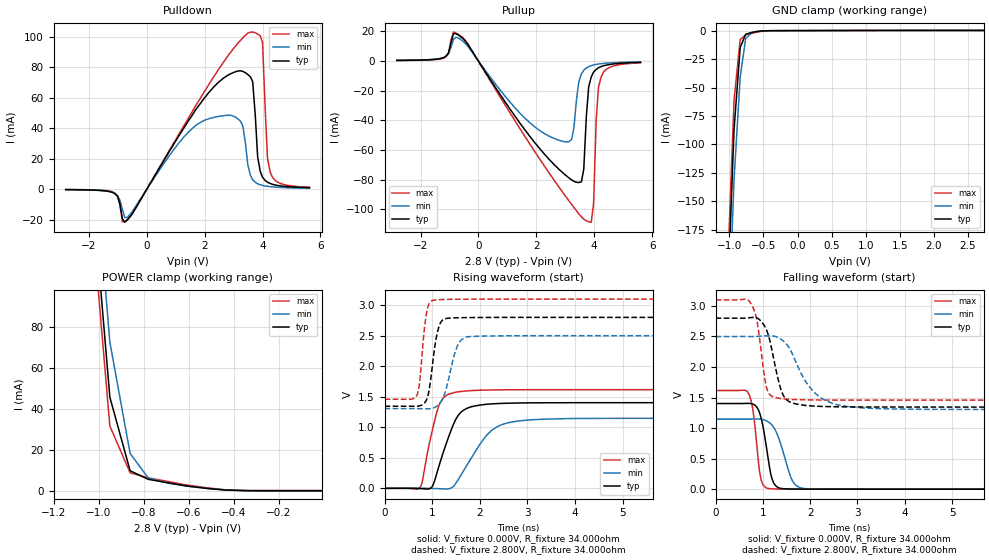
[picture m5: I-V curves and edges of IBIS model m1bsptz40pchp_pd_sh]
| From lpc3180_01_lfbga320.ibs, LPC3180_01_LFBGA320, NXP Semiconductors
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| |   Rev 0.20 IBIS Model Design Automation Generation   |
| |   N O N - S I L I C O N   C O R R E L A T E D   |
| |   This IBIS [Model] is pre-Beta tactical support   |
| |  Note: this IBIS [Model] contains clamp curves generated   |
| |   through simulation which should not be relied upon   |
| mem1bsptz40pchp
|   Bidirectional Pad 2.8
|   3state Output
|   Plain Input
|   1ns Slew Rate control
|   CMOS
| Pull Down Mode (p1=1, p2=1)
[Model]   m1bsptz40pchp_pd_sh | of mem1bsptz40pchp
Model_type   I/O
Polarity   Non-Inverting
Enable   Active-Low
|  Reciever Thresholds
Vinl   = 0.36V
Vinh   = 0.84V
| AC Test Load Conditions
Vref   = 0
Cref   = 1.2e-11
Rref   = 1000000000
Vmeas   = 0.6
| [Process Range]   typical   min   max
| C_comp edge width   400.000ps   400.000ps   400.000ps
| C_comp Tstrobe   40.000fs   40.000fs   40.000fs
C_comp   2.018pF   1.943pF   2.108pF
[Temperature Range]   25   125   -40
[Voltage Range]   2.80V   2.50V   3.10V
[GND Clamp Reference]   0.00V   0.00V   0.00V
[Pulldown Reference]   0.00V   0.00V   0.00V
[POWER Clamp Reference]   2.80V   2.50V   3.10V
[Pullup Reference]   2.80V   2.50V   3.10V
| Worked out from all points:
|   slope of the pulldown table from 0 to 0.42 V, typ, clamps not added: 31 ohm
|   slope of the pullup table from 0 to 0.42 V, typ, clamps not added: 32.8 ohm
|   GND clamp passes 1 mA (typ) near -0.61 V on its own axis
|   POWER clamp passes 1 mA (typ) near -0.49 V on its own axis
|   rising waveform, V_fixture 0.000V, R_fixture 34.000ohm: 20-80 % time 380ps typ, 593ps min, 273ps max; typ from 0 V to 1.4 V
|   falling waveform, V_fixture 0.000V, R_fixture 34.000ohm: 20-80 % time 183ps typ, 282ps min, 135ps max; typ from 1.4 V to 0 V
|   rising waveform, V_fixture 2.800V, R_fixture 34.000ohm: 20-80 % time 156ps typ, 236ps min, 119ps max; typ from 1.34 V to 2.8 V
|   falling waveform, V_fixture 2.800V, R_fixture 34.000ohm: 20-80 % time 259ps typ, 551ps min, 174ps max; typ from 2.8 V to 1.34 V
[GND Clamp]
| ref voltage   0.00V   0.00V   0.00V
|   Voltage   I(typ)   I(min)   I(max)
-2.8V     -3.643A    -3.653A    -3.644A
-1.01V    -211.8mA   -255.9mA   -186.6mA
-930mV    -86.6mA    -130.6mA   -61.24mA
-840mV    -14.83mA   -40.64mA   -7.829mA
-760mV    -3.203mA   -7.088mA   -3.83mA
-670mV    -1.622mA   -1.69mA    -2.382mA
-500mV    -233.9uA   -204.7uA   -414uA
2.73V     154.6uA    78.63uA    263.6uA
[Power Clamp]   | Vtable = Vcc - Vpad
| ref voltage   2.80V   2.50V   3.10V
|   Voltage   I(typ)   I(min)   I(max)
-2.82V    3.531A     3.518A     3.546A
-1.03V    149.7mA    178.4mA    134.4mA
-950mV    45.73mA    72.62mA    31.68mA
-860mV    9.888mA    18.31mA    8.901mA
-780mV    5.742mA    6.415mA    6.476mA
-690mV    3.983mA    3.877mA    4.635mA
-610mV    2.503mA    2.443mA    2.981mA
-440mV    510.7uA    586.4uA    642.9uA
-270mV    156.9uA    89.28uA    264.9uA
-10mV     154.6uA    73.24uA    264uA
[Pulldown]
| ref voltage   0.00V   0.00V   0.00V
|   Voltage   I(typ)   I(min)   I(max)
-2.8V     -319.3uA   -345.4uA   -253.1uA
-1.18V    -2.159mA   -2.186mA   -1.786mA
-670mV    -20.28mA   -18.52mA   -19.91mA
1.11V     35.01mA    30.34mA    36.12mA
2.13V     63.07mA    46.11mA    68.26mA
3.24V     77.61mA    44.53mA    97.58mA
3.66V     70.35mA    6.093mA    103mA
3.83V     21.24mA    3.51mA     101.7mA
4V        7.762mA    2.426mA    96.16mA
4.17V     4.525mA    1.839mA    20.54mA
4.26V     3.73mA     1.638mA    11.44mA
5.62V     952.8uA    583.3uA    1.27mA
[Pullup]   | Vtable = Vcc - Vpad
| ref voltage   2.80V   2.50V   3.10V
|   Voltage   I(typ)   I(min)   I(max)
-2.82V    285.7uA    306.1uA    228.4uA
-520mV    14.73mA    12.99mA    15.29mA
2.79V     -73.12mA   -53.48mA   -85.2mA
3.22V     -80.05mA   -52.98mA   -96.52mA
3.47V     -81.85mA   -13.92mA   -103mA
3.64V     -72.85mA   -6.25mA    -106.5mA
3.81V     -17.56mA   -3.872mA   -108.3mA
3.9V      -10.74mA   -3.234mA   -108.5mA
3.98V     -7.509mA   -2.77mA    -95.67mA
4.07V     -5.754mA   -2.418mA   -39.4mA
4.24V     -3.885mA   -1.924mA   -10.82mA
5.6V      -1.045mA   -712.7uA   -1.372mA
[Ramp]
R_load   = 34.000ohm
|   dV/dt(typ)   dV/dt(min)   dV/dt(max)
dV/dt_r   971.563mV/345.000ps   808.878mV/540.000ps   1.110V/250.000ps
dV/dt_f   1.001V/235.000ps   840.880mV/470.000ps   1.123V/165.000ps
[Rising Waveform]  | cubic spline decimation from 2001 points
V_fixture   = 0.000V
R_fixture   = 34.000ohm
|   Time   V(typ)   V(min)   V(max)
0s        4.292nV    139.7nV    2.459nV
750ps     -4.658mV   315.5uV    23.5mV
995ps     24.02mV    -2.306mV   924.1mV
1.13ns    332.7mV    -5.781mV   1.332V
1.25ns    630.1mV    -10.44mV   1.493V
1.465ns   1.081V     49.96mV    1.568V
1.715ns   1.304V     359.7mV    1.594V
2.16ns    1.377V     882.3mV    1.609V
2.675ns   1.395V     1.086V     1.614V
10ns      1.402V     1.147V     1.615V
[Falling Waveform]  | cubic spline decimation from 2001 points
V_fixture   = 0.000V
R_fixture   = 34.000ohm
|   Time   V(typ)   V(min)   V(max)
0s        1.402V     1.147V     1.615V
710ps     1.404V     1.147V     1.543V
795ps     1.389V     1.148V     1.258V
940ps     1.224V     1.146V     235.2mV
1.11ns    503.6mV    1.103V     11.61mV
1.185ns   188.3mV    1.055V     6.088mV
1.275ns   52.74mV    947.6mV    3.315mV
1.615ns   2.497mV    151.5mV    628.4uV
1.84ns    962.6uV    14.59mV    276.8uV
10ns      119.7nV    382.8nV    76.69nV
[Rising Waveform]  | cubic spline decimation from 2001 points
V_fixture   = 2.800V
V_fixture_min = 2.500V
V_fixture_max = 3.100V
R_fixture   = 34.000ohm
|   Time   V(typ)   V(min)   V(max)
0s        1.344V     1.305V     1.458V
675ps     1.344V     1.305V     1.518V
735ps     1.351V     1.304V     1.733V
830ps     1.39V      1.301V     2.572V
890ps     1.467V     1.301V     2.904V
1.045ns   2.27V      1.323V     3.083V
1.215ns   2.754V     1.458V     3.092V
1.53ns    2.793V     2.332V     3.096V
1.735ns   2.796V     2.479V     3.097V
10ns      2.799V     2.499V     3.099V
[Falling Waveform]  | cubic spline decimation from 2001 points
V_fixture   = 2.800V
V_fixture_min = 2.500V
V_fixture_max = 3.100V
R_fixture   = 34.000ohm
|   Time   V(typ)   V(min)   V(max)
0s        2.799V     2.499V     3.099V
735ps     2.808V     2.499V     3.051V
870ps     2.804V     2.501V     2.772V
1.085ns   2.59V      2.51V      1.639V
1.315ns   1.819V     2.484V     1.491V
1.435ns   1.529V     2.423V     1.479V
1.58ns    1.424V     2.279V     1.47V
2.045ns   1.362V     1.617V     1.461V
2.675ns   1.348V     1.366V     1.458V
10ns      1.344V     1.305V     1.458V
